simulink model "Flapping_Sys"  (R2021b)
settings: Solver=FixedStepAuto  StartTime=0.0  StopTime=T_s  FixedStep=1e-6  MaxStep=1e-5  RelTol=1e-6  EnableMultiTasking=on
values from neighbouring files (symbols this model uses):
  Ang_beta = 40    [Flapping_Sys_m.m]
  bm = 3.6e-6    (= 3.6e-06)    [Flapping_Sys_m.m]
  D_wing = 0.5*rho*5.35e-8    (= 3.276875e-08)    [Flapping_Sys_m.m]
  H = Radius/tan(Ang_beta*2*pi/360)    [Flapping_Sys_m.m]
  J = 2.4e-10; 1.77e-10    [Flapping_Sys_m.m]
  J0 = 7.205e-8    (= 7.205e-08)    [Flapping_Sys_m.m]
  Jg = 1e-10    [Flapping_Sys_m.m]
  K_w = J0*(Para*2*pi)^2    [Flapping_Sys_m.m]
  Ke = Kt    (= 0.01)    [Flapping_Sys_m.m]
  Kt = 1.0e-2    (= 0.01)    [Flapping_Sys_m.m]
  L = 29e-6    (= 2.9e-05)    [Flapping_Sys_m.m]
  L_wing = 0.5*rho*1.3045e-6    (= 7.9900625e-07)    [Flapping_Sys_m.m]
  ng = 25    [Flapping_Sys_m.m]
  Ra = 9    [Flapping_Sys_m.m]
  Radius = 5e-3    (= 0.005)    [Flapping_Sys_m.m]
  ur = 2.4e-3    (= 0.0024)    [Flapping_Sys_m.m]
undefined symbols (not defined in the file or in its folder): Para, Vs

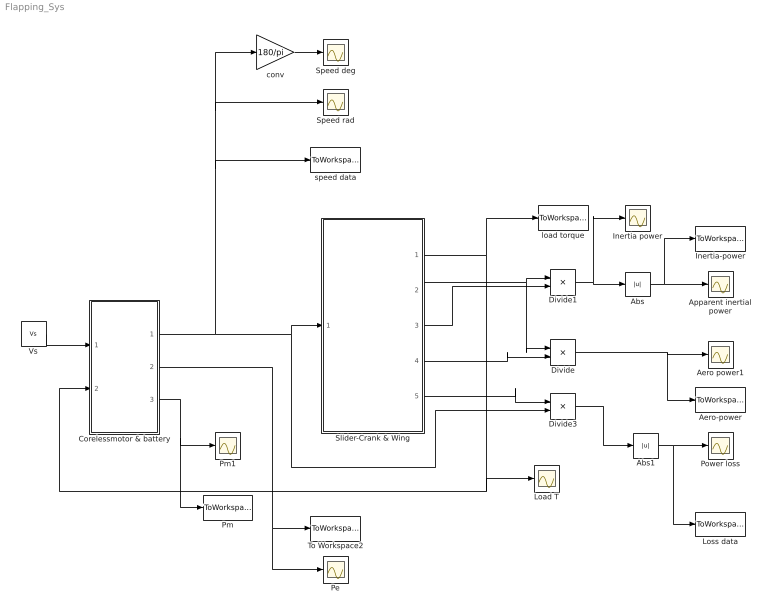
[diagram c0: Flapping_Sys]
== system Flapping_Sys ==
  Abs : Abs
  Abs1 : Abs
  Aero power1 : Scope
  Aero-power : ToWorkspace  VariableName=P_aero  SaveFormat=Timeseries  SampleTime=-1
  Apparent inertial power : Scope
  Corelessmotor & battery : Subsystem
  Divide : Product  Inputs=**
  Divide1 : Product  Inputs=**
  Divide3 : Product  Inputs=**
  Inertia power : Scope
  Inertia-power : ToWorkspace  VariableName=P_inertial  SaveFormat=Timeseries  SampleTime=-1
  Load T : Scope
  Loss data : ToWorkspace  VariableName=P_loss_cal  SaveFormat=Timeseries  SampleTime=-1
  Pe : Scope
  Pm : ToWorkspace  VariableName=Pm  SaveFormat=Timeseries  SampleTime=-1
  Pm1 : Scope
  Power loss : Scope
  Slider-Crank & Wing : Subsystem
  Speed deg : Scope
  Speed rad : Scope
  To Workspace2 : ToWorkspace  VariableName=Pe  SaveFormat=Timeseries  SampleTime=-1
  Vs : Constant  Value=Vs
  conv : Gain  Gain=180/pi
  load torque : ToWorkspace  VariableName=T_L  SaveFormat=Timeseries  SampleTime=-1
  speed data : ToWorkspace  VariableName=Speed  SaveFormat=Timeseries  SampleTime=-1
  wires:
  Corelessmotor & battery/1(W) -> conv/1, Speed rad/1, speed data/1, Slider-Crank & Wing/1(W), Divide3/2
  Vs/1 -> Corelessmotor & battery/1(Input V)
  Slider-Crank & Wing/1(T_L) -> load torque/1, Corelessmotor & battery/2(Load_T), Load T/1
  Slider-Crank & Wing/3(Reactive moment) -> Divide1/2
  Divide1/1 -> Inertia power/1, Abs/1
  Abs/1 -> Inertia-power/1, Apparent inertial power/1
  Corelessmotor & battery/2(Pe) -> Pe/1, To Workspace2/1
  Corelessmotor & battery/3(Motor power) -> Pm1/1, Pm/1
  Slider-Crank & Wing/4(aero moment) -> Divide/2
  Divide/1 -> Aero power1/1, Aero-power/1
  Slider-Crank & Wing/2(beta_dot) -> Divide/1, Divide1/1
  Slider-Crank & Wing/5(friction torque) -> Divide3/1
  Divide3/1 -> Abs1/1
  conv/1 -> Speed deg/1
  Abs1/1 -> Power loss/1, Loss data/1

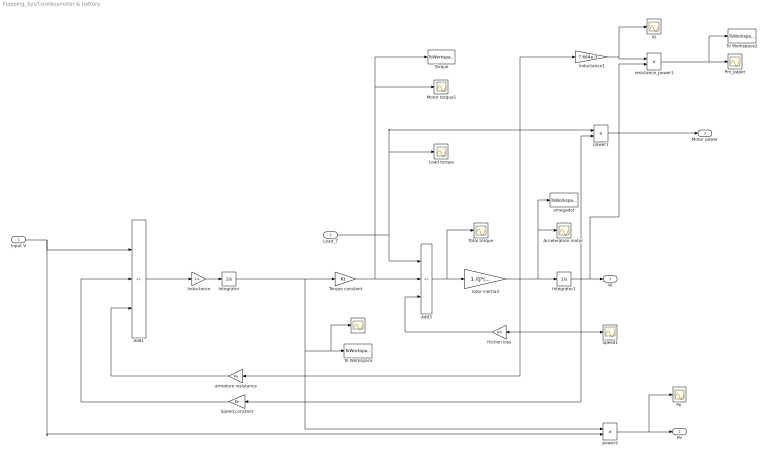
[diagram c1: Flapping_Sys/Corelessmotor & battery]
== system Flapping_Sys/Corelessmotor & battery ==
  Input V : Inport
  Load_T : Inport  Port=2
  "Acceleration motor " : Scope
  Add1 : Sum  Inputs=+--
  Add3 : Sum  Inputs=-+-
  I : Scope
  Inductance : Gain  Gain=1/L
  Inductance1 : Gain  Gain=7.664e-3
  Integrator : Integrator
  Integrator1 : Integrator
  KI : Scope
  Load torque : Scope
  Motor torque1 : Scope
  "Pe " : Scope
  Pm_paper : Scope
  Speed constant : Gain  Gain=Ke
  Speed1 : Scope
  To Workspace : ToWorkspace  VariableName=Current  SaveFormat=Timeseries  SampleTime=-1
  To Workspace2 : ToWorkspace  VariableName=KmIW  SaveFormat=Timeseries  SampleTime=-1
  Torque : ToWorkspace  VariableName=Torque  SaveFormat=Timeseries  SampleTime=-1
  Torque constant : Gain  Gain=Kt
  Total torque : Scope
  armature resistance : Gain  Gain=Ra
  friction loss : Gain  Gain=bm
  omegadot : ToWorkspace  VariableName=omegadot  SaveFormat=Timeseries  SampleTime=-1
  power1 : Product  Inputs=**
  power2 : Product  Inputs=**
  resistance_power1 : Product  Inputs=**
  rotor inertia3 : Gain  Gain=1 /(J*(ng^2)+(Jg))
  W : Outport  VectorParamsAs1DForOutWhenUnconnected=off
  Pe : Outport  Port=2  VectorParamsAs1DForOutWhenUnconnected=off
  Motor power : Outport  Port=3  VectorParamsAs1DForOutWhenUnconnected=off
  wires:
  Add1/1 -> Inductance/1
  Inductance/1 -> Integrator/1
  Input V/1 -> power2/2, Add1/1
  armature resistance/1 -> Add1/3
  friction loss/1 -> Add3/3
  Torque constant/1 -> Motor torque1/1, Torque/1, Add3/2
  Integrator1/1 -> power1/2, Speed1/1, Speed constant/1, friction loss/1, resistance_power1/2, W/1
  Load_T/1 -> power1/1, Load torque/1, Add3/1
  Add3/1 -> rotor inertia3/1, Total torque/1
  power1/1 -> Motor power/1
  Integrator/1 -> Torque constant/1, I/1, To Workspace/1, Inductance1/1, power2/1, armature resistance/1
  Inductance1/1 -> KI/1, resistance_power1/1
  resistance_power1/1 -> To Workspace2/1, Pm_paper/1
  rotor inertia3/1 -> Integrator1/1, omegadot/1, "Acceleration motor "/1
  Speed constant/1 -> Add1/2
  power2/1 -> "Pe "/1, Pe/1

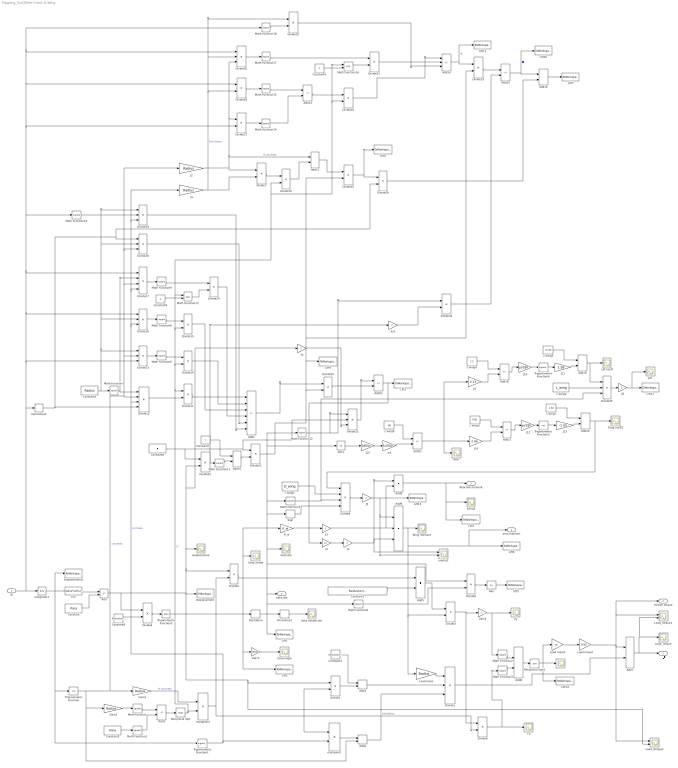
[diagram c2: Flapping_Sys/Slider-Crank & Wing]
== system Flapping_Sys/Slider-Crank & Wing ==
  W : Inport
  2y : Gain  Gain=2
  2y1 : Gain  Gain=2
  "AOA " : Scope
  Abs : Abs
  Abs1 : Abs
  Add : Sum  Inputs=+-
  Add{1,11,13,17..18} (5 alike) : Sum  Inputs=-+
  Add{3..8,10,12,16,19..20} (11 alike) : Sum
  Add14 : Sum  Inputs=+--
  Add15 : Sum  Inputs=+-
  Add2 : Sum  Inputs=++--+-
  Add21 : Sum  Inputs=+-
  Add9 : Sum  Inputs=+++
  Constant : Constant  Value=Para
  Constant1 : Constant  Value=Radius/tan(Ang_beta*2*pi/360)
  Constant2 : Constant  Value=Para
  Constant3 : Constant  Value=Radius/tan(Ang_beta*2*pi/360)
  Constant4 : Constant  Value=3
  Constant5 : Constant  Value=Radius
  Constant6 : Constant  Value=H
  Constant7 : Constant
  Constant8 : Constant  Value=Radius/tan(Ang_beta*2*pi/360)
  Constant9 : Constant  Value=3
  Derivative : Derivative
  Derivative1 : Derivative
  Derivative2 : Derivative
  Displacement : ToWorkspace  VariableName=Displacement  SaveFormat=Timeseries  SampleTime=-1
  Displacement1 : ToWorkspace  VariableName=Theta  SaveFormat=Timeseries  SampleTime=-1
  Divide1 : Product  Inputs=*/*
  Divide{2,5..7,9..11,14..15,21,24,26..29,31..32,34} (18 alike) : Product  Inputs=**
  Divide12 : Product  Inputs=****
  Divide{13,16,18..19,30,35} (6 alike) : Product  Inputs=***
  Divide17 : Product  Inputs=****
  Divide{4,20,25,33} (4 alike) : Product  Inputs=*/
  Divide22 : Product  Inputs=/*
  Divide23 : Product  Inputs=*/*
  Divide3 : Product  Inputs=/*
  Divide8 : Product  Inputs=****
  Drag coeff1 : Scope
  F : Scope
  Fcn : Fcn  Expr=Radius*sin(u(1))+sqrt(Para^2-Radius^2*(cos(u(1)))^2)
  Fx : Scope
  Fy : Scope
  Gain1 : Gain  Gain=180/pi
  Gain2 : Gain  Gain=Radius
  Gain3 : Gain  Gain=Radius
  Gain4 : Gain  Gain=-1
  Integrator1 : Integrator
  J0 : Gain  Gain=J0
  J{1,3,5,8} (4 alike) : Gain  Gain=2
  J10 : Gain  Gain=pi/180
  J11 : Gain  Gain=1.58
  J12 : Gain  Gain=pi/180
  J13 : Gain  Gain=-1.55
  J14 : Gain  Gain=2.04
  J15 : Gain  Gain=180/pi
  J2 : Gain  Gain=Radius
  J4 : Gain  Gain=Radius
  J9 : Gain  Gain=2.13
  K_w : Gain  Gain=K_w
  "Lift " : Scope
  Lift coeff : Scope
  Lift1 : ToWorkspace  VariableName=beta_dot  SaveFormat=Timeseries  SampleTime=-1
  Lift10 : ToWorkspace  VariableName=H_value  SaveFormat=Timeseries  SampleTime=-1
  Lift11 : ToWorkspace  VariableName=B_value  SaveFormat=Timeseries  SampleTime=-1
  Lift12 : ToWorkspace  VariableName=Lift  SaveFormat=Timeseries  SampleTime=-1
  Lift13 : ToWorkspace  VariableName=Drag  SaveFormat=Timeseries  SampleTime=-1
  Lift14 : ToWorkspace  VariableName=Force_h  SaveFormat=Timeseries  SampleTime=-1
  Lift2 : ToWorkspace  VariableName=beta  SaveFormat=Timeseries  SampleTime=-1
  Lift3 : ToWorkspace  VariableName=beta_Ddot  SaveFormat=Timeseries  SampleTime=-1
  Lift4 : ToWorkspace  VariableName=M_Reactive  SaveFormat=Timeseries  SampleTime=-1
  Lift5 : ToWorkspace  VariableName=Cube_beta_dot  SaveFormat=Timeseries  SampleTime=-1
  Lift6 : ToWorkspace  VariableName=M_Aero  SaveFormat=Timeseries  SampleTime=-1
  Lift7 : ToWorkspace  VariableName=beta_Ddot_1  SaveFormat=Timeseries  SampleTime=-1
  Lift8 : ToWorkspace  VariableName=I_value  SaveFormat=Timeseries  SampleTime=-1
  Lift9 : ToWorkspace  VariableName=E_value  SaveFormat=Timeseries  SampleTime=-1
  Load mass : Gain  Gain=Radius
  Load mass1 : Gain  Gain=ur
  Load mass2 : Gain  Gain=0.95
  Load_Torque : Scope
  Load_Torque1 : Scope  NumInputPorts=2
  Load_Torque2 : Scope  NumInputPorts=2
  Math Function{,1..12,14..15,17..18} (17 alike) : Math  Operator=square  SignedPower=on
  Math Function13 : Math  Operator=pow  SignedPower=on
  Math Function16 : Math  Operator=pow  SignedPower=on
  Reciprocal Sqrt : Sqrt  Operator=rSqrt
  Reciprocal Sqrt1 : Sqrt
  Sign : Signum
  Trigonometric Function : Trigonometry  Operator=cos
  Trigonometric Function1 : Trigonometry
  Trigonometric Function2 : Trigonometry  Operator=atan
  Trigonometric Function3 : Trigonometry  Operator=cos
  Trigonometric Function4 : Trigonometry
  Wing moment : Scope
  "beta double dot " : Scope
  beta angle : Scope
  beta dot : Scope
  beta_scope : Scope
  c wing1 : Constant  Value=D_wing
  c wing2 : Constant  Value=L_wing
  c wing3 : Constant  Value=9.82
  c wing4 : Constant  Value=7.2
  c wing5 : Constant  Value=0.225
  c wing7 : Constant  Value=1.92
  c wing9 : Constant  Value=90
  displacement : Scope
  inertia : Scope
  inertia1 : Scope  NumInputPorts=2
  multiplier1 : Product  Inputs=**
  multiplier2 : Product  Inputs=**
  wx : Gain  Gain=5/1000
  T_L : Outport  VectorParamsAs1DForOutWhenUnconnected=off
  beta_dot : Outport  Port=2  VectorParamsAs1DForOutWhenUnconnected=off
  Reactive moment : Outport  Port=3  VectorParamsAs1DForOutWhenUnconnected=off
  aero moment : Outport  Port=4  VectorParamsAs1DForOutWhenUnconnected=off
  friction torque : Outport  Port=5  VectorParamsAs1DForOutWhenUnconnected=off
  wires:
  Constant8/1 -> Divide4/2
  Fcn/1 -> Add/1
  Constant/1 -> Add/2
  Integrator1/1 -> Displacement1/1, Fcn/1, Trigonometric Function1/1, Trigonometric Function/1
  Derivative1/1 -> "beta double dot "/1
  Divide4/1 -> Trigonometric Function2/1
  Load mass/1 -> Divide1/1
  Divide1/1 -> Add7/2
  Gain3/1 -> Math Function/1
  Add1/1 -> Reciprocal Sqrt/1
  Gain2/1 -> multiplier2/1  "R cos theta"
  Constant2/1 -> Math Function1/1
  Reciprocal Sqrt/1 -> Math Function16/1, Divide29/2, Divide10/2, Math Function13/1, Divide15/2, Divide14/2, Divide11/1, multiplier2/2  "D"
  Trigonometric Function/1 -> Divide18/3, J2/1, Divide17/3, Divide13/2, Divide12/2, Gain2/1, Gain3/1, Add4/2  "cos theta"
  Math Function/1 -> Add1/1
  Math Function1/1 -> Add1/2
  multiplier2/1 -> Divide2/2, Divide6/2, multiplier1/1, Divide5/2  "Tan(talpha)"
  Trigonometric Function1/1 -> Divide16/3, J4/1, Divide19/3, Divide17/4, Divide12/3, multiplier1/2  "sin theta"
  Add3/1 -> Divide1/2
  multiplier1/1 -> Add4/1
  Add4/1 -> Divide1/3
  Gain1/1 -> beta angle/1
  Constant1/1 -> Add5/2
  Add5/1 -> Divide3/1
  Divide5/1 -> Add5/1
  Gain4/1 -> Fy/1, Math Function2/1
  Divide6/1 -> Fx/1, Math Function3/1
  Add6/1 -> Reciprocal Sqrt1/1
  Math Function3/1 -> Add6/2
  Math Function2/1 -> Add6/1
  Reciprocal Sqrt1/1 -> Lift14/1, Load mass1/1, F/1
  Load mass1/1 -> Load mass2/1
  Add7/1 -> T_L/1, Load_Torque/1, Load_Torque1/2
  Add8/1 -> Lift4/1, inertia/1, Reactive moment/1
  W/1 -> Derivative2/1, Divide27/2, Divide30/1, Math Function18/1, Divide28/1, Math Function10/1, Divide17/1, Divide16/1, Divide13/3, Integrator1/1
  Add9/1 -> aero moment/1, Lift6/1, Load mass/1, Divide3/2, Wing moment/1
  K_w/1 -> J3/1
  Divide3/1 -> Gain4/1, Divide6/1
  Derivative/1 -> Divide9/1, Abs1/1, Math Function12/1, Math Function4/1, Sign/1, beta dot/1, beta_dot/1, Math Function5/1, Lift1/1, Derivative1/1
  J0/1 -> J1/1
  J3/1 -> Add8/2, Add9/2
  Add/1 -> Divide4/1, 2y/1, Divide22/2, displacement/1, Divide5/1, Load_Torque2/2, Divide2/1, Displacement/1
  Constant3/1 -> Add3/1
  Divide2/1 -> Add3/2
  Sign/1 -> Divide8/4
  Abs/1 -> Lift5/1
  Divide9/1 -> Abs/1
  Math Function5/1 -> Divide9/2
  Trigonometric Function2/1 -> K_w/1, beta_scope/1, Lift2/1, Gain1/1, Derivative/1
  J1/1 -> Add8/1, Add9/3, inertia1/1
  Math Function4/1 -> Divide35/3, Divide8/3
  Constant5/1 -> Divide19/1, Divide18/2, Divide16/2, Divide13/1, Math Function7/1
  Divide12/1 -> Divide11/2
  Divide11/1 -> Add2/1
  Math Function7/1 -> Divide17/2, Divide12/1
  Divide13/1 -> Math Function6/1
  Math Function6/1 -> Divide14/1
  Divide14/1 -> Add2/2
  Math Function8/1 -> Divide15/1
  Divide16/1 -> Math Function8/1
  Divide15/1 -> Add2/3
  Derivative2/1 -> Divide26/2, Divide18/1, Divide12/4
  Divide17/1 -> Math Function9/1
  Divide18/1 -> Add2/5
  Math Function10/1 -> Divide19/2
  Divide19/1 -> Add2/6
  Add2/1 -> Divide20/1
  Constant6/1 -> Divide22/1, Divide21/1, Divide23/2
  Add10/1 -> Divide21/2
  Constant7/1 -> Add10/1
  Divide22/1 -> 2y1/1, Math Function11/1
  Math Function11/1 -> Add10/2
  Divide21/1 -> Divide25/2, Divide33/2, Lift9/1, Divide20/2  "E"
  Divide20/1 -> Add11/2
  Math Function12/1 -> Divide34/1, Divide23/1
  Divide23/1 -> Add11/1
  Add11/1 -> J0/1, Lift3/1
  2y/1 -> Divide23/3
  Constant9/1 -> Math Function13/2
  Math Function9/1 -> Divide24/1
  Math Function13/1 -> Divide24/2
  Divide24/1 -> Add2/4
  J2/1 -> Divide30/3, Divide27/1, Add12/1, Divide7/1  "R cos theta"
  J4/1 -> Divide30/2, Divide32/1, Divide28/2, Divide7/2  "R sin theta"
  Divide7/1 -> Divide10/1
  Divide10/1 -> Add12/2
  Add12/1 -> Divide25/1
  Divide25/1 -> Lift8/1, Divide26/1  "I"
  Divide27/1 -> Math Function14/1
  Divide28/1 -> Math Function15/1
  Math Function15/1 -> Add13/1
  Math Function14/1 -> Add13/2
  Add13/1 -> Divide29/1
  Constant4/1 -> Math Function16/2
  Divide30/1 -> Math Function17/1
  Math Function16/1 -> Divide31/2
  Math Function17/1 -> Divide31/1
  Divide31/1 -> Add14/2
  Divide29/1 -> Add14/1
  Math Function18/1 -> Divide32/2
  Divide32/1 -> Add14/3
  Add14/1 -> Lift11/1, Divide33/1  "B"
  Divide33/1 -> Add15/1
  2y1/1 -> Divide34/2
  Divide34/1 -> Add15/2
  Divide26/1 -> Add16/2
  Add15/1 -> Lift10/1, Add16/1  "H"
  Add16/1 -> Lift7/1
  c wing1/1 -> Divide8/2
  J5/1 -> Add9/1, inertia1/2, Lift13/1
  Divide8/1 -> J5/1
  Divide35/1 -> J8/1
  J8/1 -> "Lift "/1, Lift12/1
  J9/1 -> Add18/2
  c wing4/1 -> Add18/1
  c wing5/1 -> Add19/1
  Trigonometric Function4/1 -> J11/1
  Add19/1 -> Lift coeff/1, Divide35/1
  J11/1 -> Add19/2
  Add18/1 -> J10/1
  J10/1 -> Trigonometric Function4/1
  c wing2/1 -> Divide35/2
  J12/1 -> Trigonometric Function3/1
  Add17/1 -> J12/1
  Add21/1 -> "AOA "/1, J9/1, J14/1
  J13/1 -> Add20/2
  Add20/1 -> Drag coeff1/1, Divide8/1
  Trigonometric Function3/1 -> J13/1
  c wing7/1 -> Add20/1
  c wing3/1 -> Add17/1
  J14/1 -> Add17/2
  J15/1 -> wx/1
  c wing9/1 -> Add21/1
  wx/1 -> Add21/2
  Abs1/1 -> J15/1
  Load mass2/1 -> Load_Torque2/1, friction torque/1, Load_Torque1/1, Add7/1
